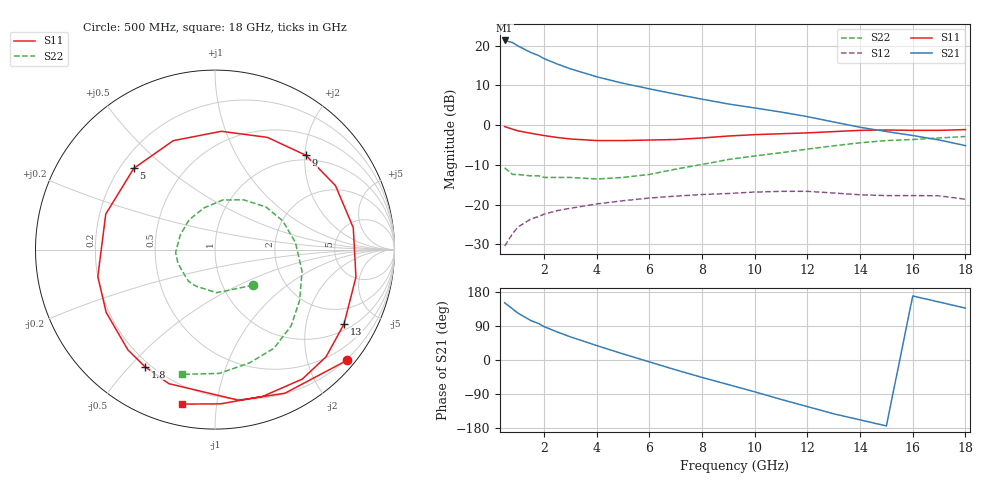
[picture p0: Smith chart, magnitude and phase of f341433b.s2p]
!ATF-34143
!S-PARAMETERS at Vds=3V  Id=40mA.  LAST UPDATED 01-29-99
# ghz s ma r 50
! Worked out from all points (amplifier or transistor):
!   23 points, 500 MHz to 18 GHz, reference 50 ohm
!   highest |S21| = 21.3 dB at 500 MHz (marker M1)
!   |S21| within 3 dB of that: start of sweep to 1.489 GHz
!   unconditionally stable (mu >= 1): 5.776 GHz to end of sweep
!   at 1.5 GHz: K = 0.42, MSG = 20.9 dB, |S12| = -23.6 dB
!   at 7 GHz: K = 1.09, MAG = 11.0 dB, |S12| = -17.9 dB
!   at 18 GHz: K = 1.42, MAG = 2.9 dB, |S12| = -18.6 dB
!   lowest NFmin = 0.10 dB at 500 MHz
!   S11 on the Smith chart (normalised r, x): 500 MHz: 0.17, -2.74; 1.8 GHz: 0.18, -0.55; 5 GHz: 0.26, +0.39; 9 GHz: 0.90, +2.02; 13 GHz: 1.24, -3.30; 18 GHz: 0.11, -0.80
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0.5  0.96 -40.0  11.64 151.0  0.03 68.0  0.29 -43.0
0.8  0.89 -64.0  10.95 135.0  0.043 56.0  0.24 -70.0
1  0.85 -81.0  9.956 124.0  0.052 49.0  0.24 -88.0
1.5  0.79 -109.0  8.209 104.0  0.066 36.0  0.23 -118.0
1.8  0.76 -121.0  7.495 96.0  0.071 32.0  0.23 -130.0
2  0.74 -131.0  6.876 88.0  0.076 27.0  0.22 -141.0
2.5  0.7 -150.0  5.88 74.0  0.084 19.0  0.22 -160.0
3  0.67 -167.0  5.12 61.0  0.09 12.0  0.22 -176.0
4  0.64 162.0  4.063 38.0  0.102 -1.0  0.21 157.0
5  0.64 135.0  3.365 16.0  0.112 -14.0  0.22 131.0
6  0.65 111.0  2.867 -5.0  0.121 -28.0  0.24 105.0
7  0.66 87.0  2.454 -26.0  0.128 -42.0  0.28 81.0
8  0.69 65.0  2.125 -46.0  0.134 -55.0  0.32 60.0
9  0.73 46.0  1.848 -65.0  0.138 -69.0  0.37 40.0
10  0.76 28.0  1.647 -84.0  0.144 -84.0  0.41 23.0
11  0.78 9.0  1.462 -104.0  0.147 -99.0  0.45 5.0
12  0.8 -11.0  1.281 -123.0  0.147 -114.0  0.5 -14.0
13  0.83 -30.0  1.095 -142.0  0.14 -130.0  0.55 -31.0
15  0.87 -56.0  0.831 -174.0  0.13 -154.0  0.64 -59.0
16  0.86 -72.0  0.741 169.0  0.13 -166.0  0.66 -73.0
17  0.86 -88.0  0.652 153.0  0.129 179.0  0.69 -88.0
18  0.88 -102.0  0.553 137.0  0.117 166.0  0.72 -105.0
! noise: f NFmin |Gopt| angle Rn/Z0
0.5  0.1  0.87  13  0.16
0.9  0.13  0.82  28  0.13
1.5  0.17  0.73  50  0.1
1.8  0.21  0.7  61  0.09
2.5  0.29  0.6  87  0.06
3  0.35  0.54  106  0.05
5  0.6  0.41  -178  0.03
6  0.72  0.39  -142  0.06
8  0.97  0.45  -80  0.21
10  1.22  0.61  -39  0.5
